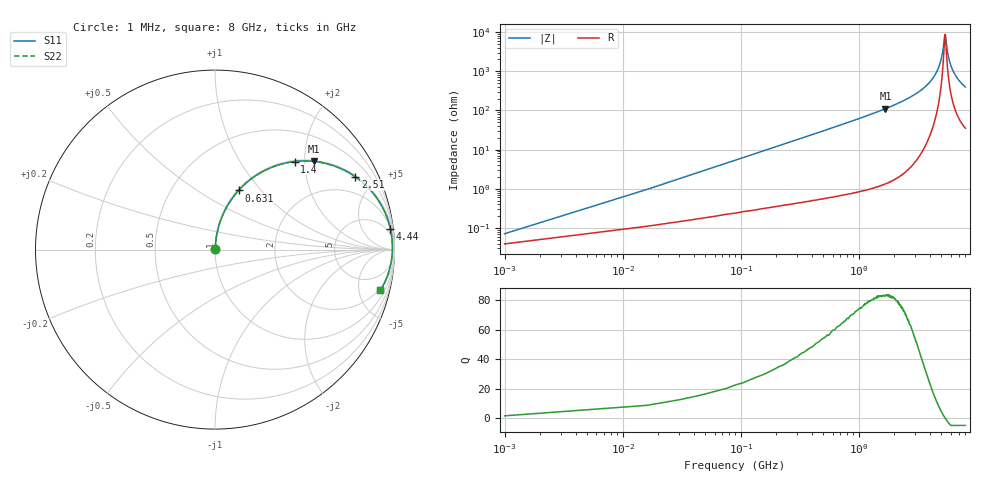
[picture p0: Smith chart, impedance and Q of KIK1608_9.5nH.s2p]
!version-2
!date-01.2022
!Series
# MHz S RI R 50
!Freq ReS11 ImS11 ReS21 ImS21 ReS12 ImS12 ReS22 ImS22
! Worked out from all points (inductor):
!   535 points, 1 MHz to 8 GHz, reference 50 ohm
!   read as one part in series: L = 9.5 nH near 31 MHz
!   highest Q = 83.3 at 1.68 GHz (marker M1), where L = 10.5 nH
!   self-resonance near 5.37 GHz
!   S11 on the Smith chart (normalised r, x): 1 MHz: 1.00, +0.00; 631 MHz: 1.01, +0.76; 1.4 GHz: 1.02, +1.79; 2.51 GHz: 1.05, +3.82; 4.44 GHz: 2, +16; 8 GHz: 1.70, -7.87
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1  0.000384 0.000596  0.9996 -0.000596  0.9996 -0.000596  0.000384 0.000596
46  0.00251 0.0273  0.9975 -0.0273  0.9975 -0.0273  0.00251 0.0273
76  0.00426 0.0451  0.9957 -0.0451  0.9957 -0.0451  0.00426 0.0451
121  0.00792 0.0715  0.9921 -0.0715  0.9921 -0.0715  0.00792 0.0715
196  0.0169 0.1148  0.9831 -0.1148  0.9831 -0.1148  0.0169 0.1148
316  0.0385 0.1812  0.9615 -0.1812  0.9615 -0.1812  0.0385 0.1812
631  0.1314 0.3296  0.8686 -0.3296  0.8686 -0.3296  0.1314 0.3296
1340  0.4203 0.4875  0.5797 -0.4875  0.5797 -0.4875  0.4203 0.4875
1400  0.4446 0.4908  0.5554 -0.4908  0.5554 -0.4908  0.4446 0.4908
1680  0.5522 0.4913  0.4478 -0.4913  0.4478 -0.4913  0.5522 0.4913
2510  0.7815 0.4061  0.2185 -0.4061  0.2185 -0.4061  0.7815 0.4061
2670  0.8135 0.3818  0.1865 -0.3818  0.1865 -0.3818  0.8135 0.3818
4010  0.9591 0.1776  0.0409 -0.1776  0.0409 -0.1776  0.9591 0.1776
4440  0.9772 0.1168  0.0228 -0.1168  0.0228 -0.1168  0.9772 0.1168
5000  0.9877 0.0457  0.0123 -0.0457  0.0123 -0.0457  0.9877 0.0457
5180  0.9887 0.0241  0.0113 -0.0241  0.0113 -0.0241  0.9887 0.0241
5340  0.9887 0.00504  0.0113 -0.00504  0.0113 -0.00504  0.9887 0.00504
5420  0.9885 -0.00343  0.0115 0.00343  0.0115 0.00343  0.9885 -0.00343
5640  0.987 -0.0281  0.013 0.0281  0.013 0.0281  0.987 -0.0281
5910  0.9837 -0.0562  0.0163 0.0562  0.0163 0.0562  0.9837 -0.0562
6680  0.967 -0.1279  0.033 0.1279  0.033 0.1279  0.967 -0.1279
8000  0.9219 -0.2273  0.0781 0.2273  0.0781 0.2273  0.9219 -0.2273
